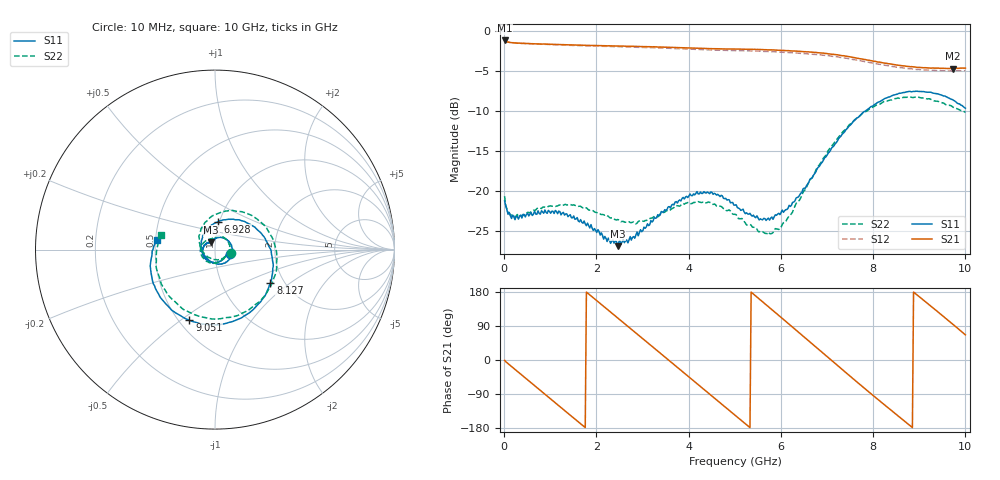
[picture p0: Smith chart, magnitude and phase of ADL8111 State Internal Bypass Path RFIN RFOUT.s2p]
! Analog Devices Inc.
! Device:  ADL8111
! Description: Bypass Amplifier
! Frequency:  0.00 -  8.00 GHz
! Package:28-Lead Lead Frame Chip Scale Package[LFCSP] 6mm by 6mm
! Conditions:	Vdd = 5.0 V
!		State: Internal Bypass
!		Path:  RFIN (Port 1) to RFOUT (Port 2)
!		Idq = 70mA
!		Pin = -10 dBm
!		Temp = +25 C (baseplate temperature)
! Freq(Hz)	S11a(dB)	S11p(deg)	S21a(dB)	S21p(deg)	S12a(dB)	S12p(deg)	S22a(dB)	S22p(deg)
# Hz S  dB  R 50
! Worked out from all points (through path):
!   401 points, 10 MHz to 10 GHz, reference 50 ohm
!   highest |S21| = -1.17 dB at 10 MHz (marker M1); lowest = -4.7 dB at 9.725 GHz (marker M2)
!   group delay of S21, straight-line fit = 282 ps
!   lowest |S11| = -26.9 dB at 2.458 GHz (marker M3), VSWR 1.09, Z = 47.7 + j3.79 ohm
!   |S11| at or under -10 dB: start of sweep to 7.834 GHz
!   |S22| runs from -25.4 to -8.2 dB; largest |S21 - S12| = 0.022
!   S11 on the Smith chart (normalised r, x): 10 MHz: 1.18, -0.05; 6.928 GHz: 0.98, +0.31; 8.127 GHz: 1.69, -0.73; 9.051 GHz: 0.56, -0.54; 10 GHz: 0.51, +0.06
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1e7  -21.23 -14.9  -1.17 -0.8  -1.22 -1.1  -20.65 -13.5
4.84525e8  -22.92 -68.4  -1.55 -50.1  -1.56 -50.0  -22.79 -70.2
8.5915e8  -22.79 -114.3  -1.61 -87.9  -1.65 -87.9  -22.00 -113.1
1.233775e9  -22.99 -155.5  -1.70 -125.6  -1.74 -125.6  -21.84 -152.3
1.683325e9  -23.91 162.2  -1.76 -170.8  -1.83 -170.8  -22.04 168.9
2.032975e9  -24.84 138.9  -1.81 154.1  -1.88 154.2  -22.74 144.6
2.45755e9  -26.91 118.6  -1.87 111.5  -1.96 111.5  -23.57 121.2
2.882125e9  -25.13 101.7  -1.92 68.7  -2.02 68.7  -24.02 104.6
3.35665e9  -23.05 72.3  -2.00 20.9  -2.11 20.8  -23.11 87.0
3.781225e9  -21.23 39.4  -2.06 -22.0  -2.19 -22.0  -21.87 64.4
4.25575e9  -20.14 -5.7  -2.15 -69.8  -2.30 -69.8  -21.41 30.0
5.005e9  -21.77 -78.7  -2.25 -145.4  -2.44 -145.4  -22.92 -32.7
5.479525e9  -23.11 -122.1  -2.29 166.3  -2.50 166.2  -24.76 -80.6
5.979025e9  -22.95 -173.6  -2.40 115.0  -2.63 115.0  -24.74 -146.7
6.678325e9  -18.36 109.7  -2.63 42.7  -2.88 42.7  -18.33 134.0
6.928075e9  -16.08 83.9  -2.75 16.8  -3.02 16.7  -15.85 110.0
7.577425e9  -11.25 19.2  -3.30 -50.6  -3.56 -50.7  -11.23 45.4
8.126875e9  -8.84 -31.3  -3.87 -106.3  -4.14 -106.5  -9.14 -8.6
8.35165e9  -8.24 -51.2  -4.08 -128.8  -4.35 -128.9  -8.65 -30.9
9.05095e9  -7.55 -109.8  -4.57 162.1  -4.84 162.0  -8.35 -100.2
9.725275e9  -8.59 -166.0  -4.69 94.7  -4.98 94.6  -9.49 -167.4
1e10  -9.64 170.7  -4.62 66.3  -4.95 66.2  -10.18 165.2
